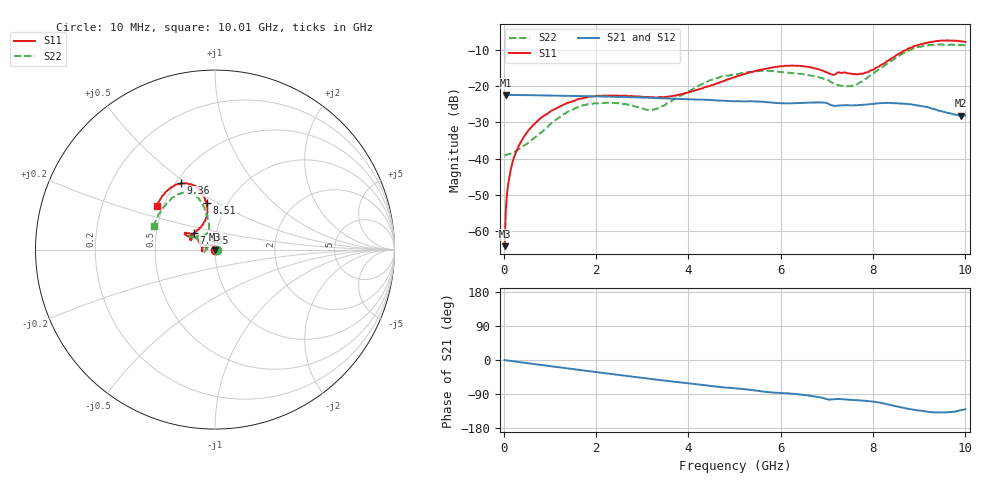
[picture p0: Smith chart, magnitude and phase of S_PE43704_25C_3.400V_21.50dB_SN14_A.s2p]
! Device ID: PE43704
! Dir: z:\PE43704\PE43704_Char_1_20130516\PE43704\AMB\3p400V\21p50dB
! Serial: 14
! Insertion: A
! Impedance: 50 ohm
! Temp: Amb
! VDD: 3.400V
! Attenuation Step: 21.50dB
! IDD: 1.139951e-01mA
#  Hz  S  RI  R  50
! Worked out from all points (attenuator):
!   401 points, 10 MHz to 10.01 GHz, reference 50 ohm
!   highest |S21| = -22.45 dB at 35 MHz (marker M1); lowest = -28.2 dB at 9.91 GHz (marker M2)
!   lowest |S11| = -64.1 dB at 10 MHz (marker M3), VSWR 1.00, Z = 50 + j0.0443 ohm
!   |S11| at or under -10 dB: start of sweep to 8.73 GHz
!   |S22| runs from -39.1 to -8.5 dB; largest |S21 - S12| = 0.00087
!   S11 on the Smith chart (normalised r, x): 10 MHz: 1.00, +0.00; 7.485 GHz: 0.78, +0.15; 8.51 GHz: 0.80, +0.45; 9.36 GHz: 0.53, +0.48; 10.01 GHz: 0.46, +0.27
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1e7  0.000438 0.000443  0.0754 -0.000197  0.0755 -0.000214  0.011 0.000347
3.5e7  0.000592 0.00179  0.0755 -0.000824  0.0755 -0.000835  0.0112 0.00119
8.5e7  0.000499 0.00433  0.0753 -0.00198  0.0753 -0.00193  0.011 0.00308
1.6e8  0.000106 0.00785  0.0752 -0.00362  0.0751 -0.00359  0.0104 0.0059
2.6e8  -0.00178 0.0122  0.0749 -0.00574  0.0749 -0.00571  0.00851 0.00945
4.35e8  -0.00617 0.0194  0.0742 -0.00938  0.0743 -0.0094  0.00384 0.0147
1.01e9  -0.034 0.0296  0.0712 -0.0209  0.0711 -0.0209  -0.0238 0.0185
1.685e9  -0.0657 0.0146  0.0649 -0.0331  0.0649 -0.033  -0.0538 -0.00147
2.26e9  -0.0735 -0.0027  0.0578 -0.0419  0.0579 -0.0418  -0.0566 -0.0156
3.36e9  -0.0704 -0.00162  0.0413 -0.054  0.0414 -0.054  -0.049 0.00779
4.41e9  -0.0882 0.0425  0.025 -0.0596  0.0249 -0.0595  -0.0968 0.0619
5.01e9  -0.1125 0.071  0.0164 -0.0596  0.0164 -0.0596  -0.1262 0.0708
5.96e9  -0.1602 0.0937  0.00337 -0.0579  0.00365 -0.058  -0.1405 0.0697
6.685e9  -0.1607 0.0794  -0.00535 -0.0589  -0.00523 -0.0589  -0.1215 0.0662
7.11e9  -0.1304 0.061  -0.0132 -0.0525  -0.0132 -0.0527  -0.0826 0.0763
7.485e9  -0.1167 0.0934  -0.0141 -0.0524  -0.0141 -0.0524  -0.0505 0.0866
7.835e9  -0.0741 0.1334  -0.0168 -0.0528  -0.0169 -0.0529  -0.0336 0.1202
8.36e9  -0.0426 0.2244  -0.0275 -0.0516  -0.0276 -0.0516  -0.0484 0.2064
8.51e9  -0.0459 0.2593  -0.031 -0.0488  -0.0305 -0.0494  -0.0608 0.2387
9.36e9  -0.1883 0.37  -0.0352 -0.0317  -0.0357 -0.0314  -0.2152 0.3048
9.91e9  -0.3064 0.2765  -0.0265 -0.0287  -0.0267 -0.0283  -0.3264 0.1683
1.001e10  -0.3239 0.2425  -0.0252 -0.0301  -0.0259 -0.0303  -0.3403 0.1293
